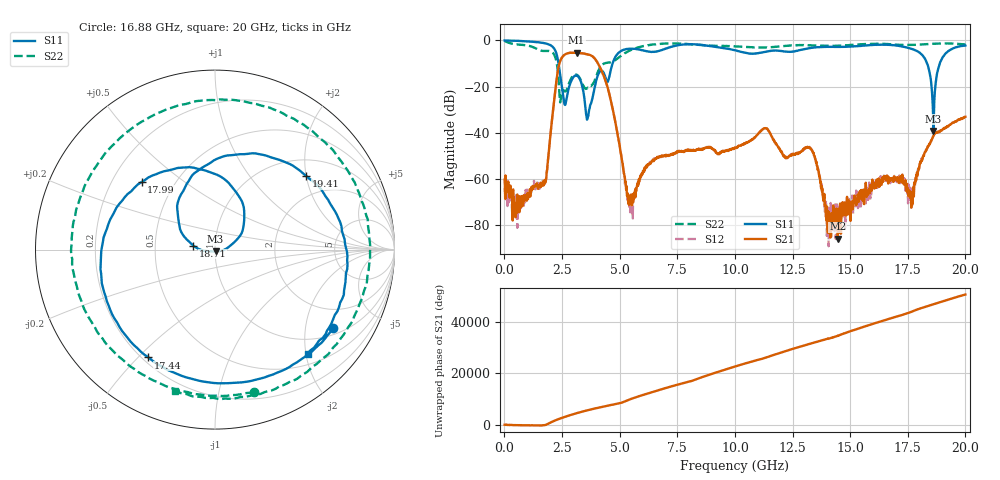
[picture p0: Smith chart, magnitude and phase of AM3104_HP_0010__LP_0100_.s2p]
!Created with skrf (http://scikit-rf.org).
# Hz S RI R 50.0
!freq ReS11 ImS11 ReS21 ImS21 ReS12 ImS12 ReS22 ImS22
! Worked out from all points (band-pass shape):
!   1601 points, 10 MHz to 20 GHz, reference 50 ohm
!   highest |S21| = -5.27 dB at 3.133 GHz (marker M1); lowest = -85.8 dB at 14.47 GHz (marker M2)
!   |S21| within 3 dB of the highest: 2.448 GHz to 3.955 GHz (1.507 GHz wide, 47.1 % of centre)
!   lowest |S11| = -39.1 dB at 18.61 GHz (marker M3), VSWR 1.02, Z = 50.3 - j1.06 ohm
!   |S11| at or under -10 dB: 2.349 GHz to 4.692 GHz (2.342 GHz wide, 66.5 % of centre); 18.34 GHz to 18.88 GHz (544.1 MHz wide, 2.92 % of centre)
!   |S22| runs from -26.8 to -0.2 dB; largest |S21 - S12| = 0.0044
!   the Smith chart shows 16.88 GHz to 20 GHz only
!   S11 on the Smith chart (normalised r, x): 16.88 GHz: 1.22, -2.83; 17.44 GHz: 0.22, -0.54; 17.99 GHz: 0.33, +0.35; 18.71 GHz: 0.78, +0.03; 19.41 GHz: 1.40, +2.00; 20 GHz: 0.69, -2.04
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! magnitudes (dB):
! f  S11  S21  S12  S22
! 10 MHz  0.0  -60.2  -64.0  -0.2
! 1.722 GHz  -1.1  -61.1  -61.6  -4.6
! 2.384 GHz  -12.3  -10.1  -10.1  -22.5
! 2.634 GHz  -27.9  -6.0  -6.0  -22.0
! 3.133 GHz  -15.2  -5.3  -5.3  -14.9
! 3.346 GHz  -18.6  -5.6  -5.5  -17.7
! 3.621 GHz  -33.0  -6.1  -6.0  -20.4
! 4.395 GHz  -16.2  -17.6  -17.6  -9.7
! 5.47 GHz  -3.6  -66.8  -70.4  -4.2
! 6.682 GHz  -4.6  -50.6  -50.6  -1.5
! 10.01 GHz  -4.2  -46.6  -46.6  -2.5
! 13.34 GHz  -3.1  -47.5  -47.3  -2.1
! 14.04 GHz  -2.8  -83.3  -84.4  -2.3
! 14.47 GHz  -2.8  -85.8  -74.5  -2.3
! 16.68 GHz  -1.8  -60.5  -58.9  -1.6
! 16.88 GHz  -2.1  -60.1  -60.1  -1.7
! 17.44 GHz  -3.0  -62.5  -62.1  -1.9
! 17.99 GHz  -5.1  -55.7  -54.9  -1.8
! 18.61 GHz  -39.1  -41.3  -41.4  -1.4
! 18.71 GHz  -18.3  -40.0  -40.0  -1.4
! 19.41 GHz  -3.7  -35.9  -35.8  -1.3
! 20 GHz  -2.2  -33.0  -32.9  -1.7
